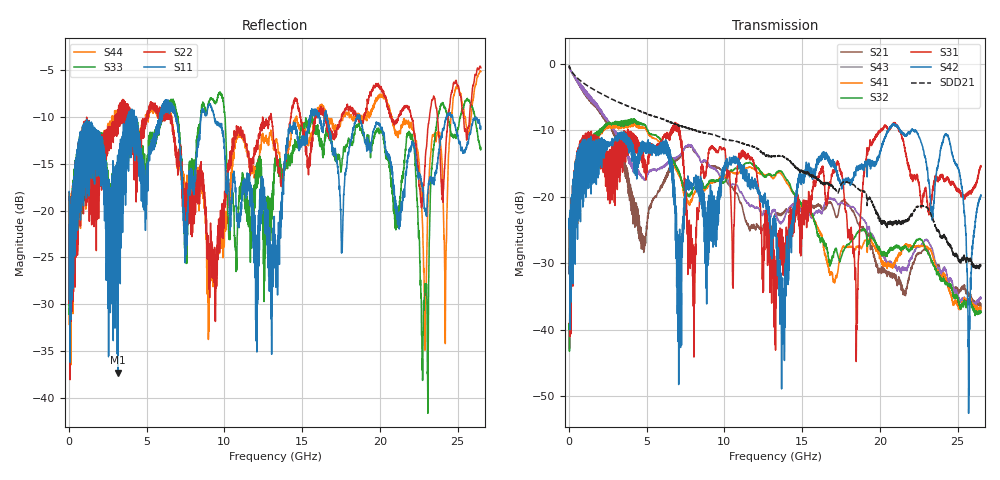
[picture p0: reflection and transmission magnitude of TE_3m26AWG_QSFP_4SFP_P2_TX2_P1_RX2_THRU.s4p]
!Agilent Technologies,N5222A,MY51421691,A.10.00.00
!Agilent N5222A: A.10.00.00
!Date: Friday, January 30, 2015 12:33:33
!Correction: S11(Full 4 Port(1,2,3,4))
!S12(Full 4 Port(1,2,3,4))
!S13(Full 4 Port(1,2,3,4))
!S14(Full 4 Port(1,2,3,4))
!S21(Full 4 Port(1,2,3,4))
!S22(Full 4 Port(1,2,3,4))
!S23(Full 4 Port(1,2,3,4))
!S24(Full 4 Port(1,2,3,4))
!S31(Full 4 Port(1,2,3,4))
!S32(Full 4 Port(1,2,3,4))
!S33(Full 4 Port(1,2,3,4))
!S34(Full 4 Port(1,2,3,4))
!S41(Full 4 Port(1,2,3,4))
!S42(Full 4 Port(1,2,3,4))
!S43(Full 4 Port(1,2,3,4))
!S44(Full 4 Port(1,2,3,4))
!S4P File: Measurements: <S11,S12,S13,S14>,
!<S21,S22,S23,S24>,
!<S31,S32,S33,S34>,
!<S41,S42,S43,S44>:
# Hz S  dB  R 50.0
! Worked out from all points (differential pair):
!   2650 points, 10 MHz to 26.5 GHz, reference 50 ohm
!   strongest paths, dB at 10 MHz, 6.63 GHz, 13.26 GHz, 19.88 GHz, 26.5 GHz:
!     S42: -24.7, -16.4, -25.3, -14.1, -19.7
!     S31: -24.9, -10.2, -30.6, -10.6, -15.3
!     S32: -39.9, -14.3, -16.8, -27.4, -37.4
!     S41: -39.5, -14.8, -16.9, -28.1, -37.1
!     S43: -0.4, -14.4, -22.1, -27.5, -35.3
!     S21: -0.4, -15.2, -22.8, -30.7, -36.5
!   taken as a pair (ports 3,1 in; 4,2 out), SDD21 dB: -0.3, -8.8, -13.9, -22.6, -30.6
!   lowest |S11| = -37.3 dB at 3.15 GHz (marker M1), VSWR 1.03, Z = 50.5 - j1.27 ohm
!   |S11| at or under -10 dB: start of sweep to 3.77 GHz; 9.339 GHz to 15.5 GHz (6.157 GHz wide, 49.6 % of centre); 18.72 GHz to 24.29 GHz (5.572 GHz wide, 25.9 % of centre)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
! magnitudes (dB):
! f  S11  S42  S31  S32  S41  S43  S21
! 10 MHz  -18.0  -24.7  -24.9  -39.9  -39.5  -0.4  -0.4
! 3.15 GHz  -37.3  -11.0  -17.0  -8.8  -9.3  -10.8  -11.7
! 13.77 GHz  -17.7  -33.8  -27.4  -16.5  -16.9  -23.6  -22.4
! 15.33 GHz  -12.1  -16.5  -23.1  -21.7  -21.6  -21.8  -20.7
! 22.9 GHz  -20.1  -14.0  -19.0  -27.6  -27.3  -26.6  -27.9
! 25.74 GHz  -12.1  -49.7  -19.3  -36.0  -35.6  -35.9  -34.9
! 26.5 GHz  -11.0  -19.7  -15.3  -37.4  -37.1  -35.3  -36.5
